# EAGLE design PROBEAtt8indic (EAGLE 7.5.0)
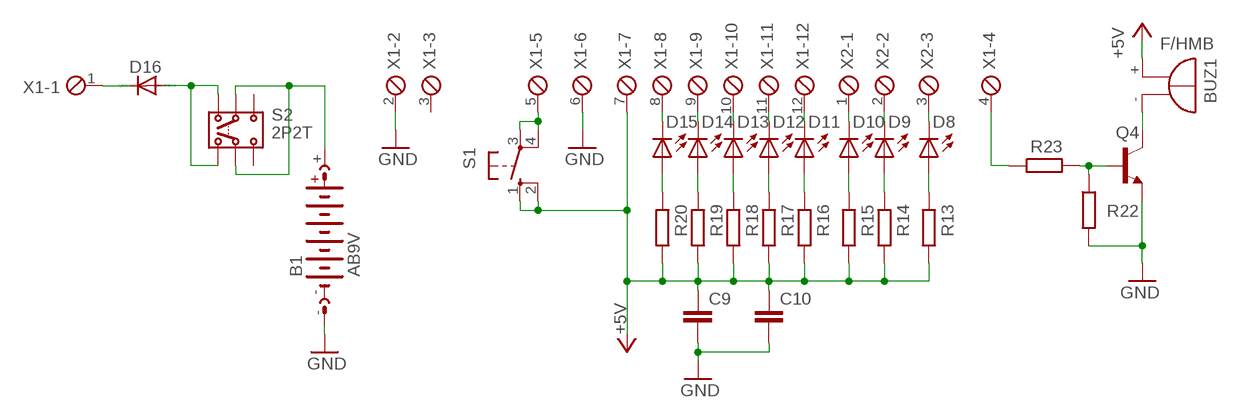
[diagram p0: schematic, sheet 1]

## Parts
B1  AB9V  [AB9V]
BUZ1  F/HMB  [F/HMB]
C9  C-EUC1206  [C1206]
C10  C-EUC1206  [C1206]
D8  LED5MM  [LED5MM]
D9  LED5MM  [LED5MM]
D10  LED5MM  [LED5MM]
D11  LED5MM  [LED5MM]
D12  LED5MM  [LED5MM]
D13  LED5MM  [LED5MM]
D14  LED5MM  [LED5MM]
D15  LED5MM  [LED5MM]
D16  1N4004  [DO41-10]
Q4  BC337  [TO92]
R13  R-EU_0204/7  [0204/7]
R14  R-EU_0204/7  [0204/7]
R15  R-EU_0204/7  [0204/7]
R16  R-EU_0204/7  [0204/7]
R17  R-EU_0204/7  [0204/7]
R18  R-EU_0204/7  [0204/7]
R19  R-EU_0204/7  [0204/7]
R20  R-EU_0204/7  [0204/7]
R22  R-EU_0204/7  [0204/7]
R23  R-EU_0204/7  [0204/7]
S1  10-XX  [B3F-10XX]
S2  2P2T  [2P2T]
X1  MPT12  [12POL254]
X2  MPT3  [3POL254]

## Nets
+5V: BUZ1.+ C9.1 C10.1 R13.1 R14.1 R15.1 R16.1 R17.1 R18.1 R19.1 R20.1 S1.1(S) S1.2(S1) X1.7
GND: B1.- C9.2 C10.2 Q4.1(E) R22.2 X1.2 X1.6
N$1: R23.1 X1.4
N$2: D8.K(C) X2.3
N$3: D9.K(C) X2.2
N$4: S1.3(P) S1.4(P1) X1.5
N$5: D10.K(C) X2.1
N$6: D16.C X1.1
N$7: D11.K(C) X1.12
N$8: D12.K(C) X1.11
N$9: Q4.2(B) R22.1 R23.2
N$10: D13.K(C) X1.10
N$11: D14.K(C) X1.9
N$12: D15.K(C) X1.8
N$13: D15.A R20.2
N$14: D14.A R19.2
N$15: D13.A R18.2
N$16: D12.A R17.2
N$17: D11.A R16.2
N$18: D10.A R15.2
N$19: D9.A R14.2
N$20: D16.A S2.1.1 S2.1.2
N$21: D8.A R13.2
N$22: B1.+ S2.2.1 S2.2.2
N$23: BUZ1.- Q4.3(C)
Unconnected: S2.3.1 S2.3.2 X1.3

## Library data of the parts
B1 = battery:AB9V: 9-V BATTERY CLIP
BUZ1 = buzzer:F/HMB: BUZZER; OC_FARNELL: unknown; OC_NEWARK: unknown
C9 C10 = rcl:C-EU: CAPACITOR, European symbol
D8-D15 = led:LED: LED
D16 = diode:1N4004: DIODE
Q4 = transistor:BC337: NPN TRANSISTOR
R13-R20 R22 R23 = rcl:R-EU_: RESISTOR, European symbol
S1 = switch-omron:10-XX: OMRON SWITCH; MPN: B3F-1000; OC_FARNELL: 176432; OC_NEWARK: 36M3542
S2 = switch:2P2T: SLIDE SWITCH 2P2T Part No. SS-22F05-G(A)4 Source: CANAL ELECTRONIC CO., LTD .. switsch.pdf
X1 = con-phoenix-254:MPT12: PHOENIX CONNECTOR; OC_FARNELL: unknown; OC_NEWARK: unknown
X2 = con-phoenix-254:MPT3: PHOENIX CONNECTOR; OC_FARNELL: unknown; OC_NEWARK: unknown

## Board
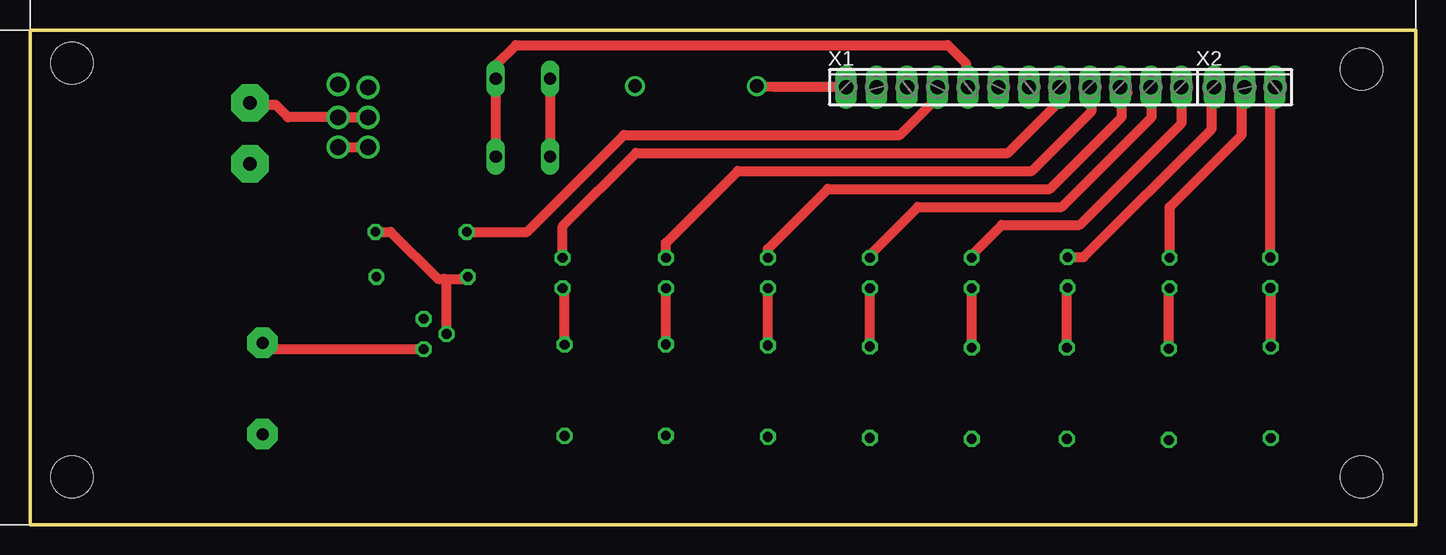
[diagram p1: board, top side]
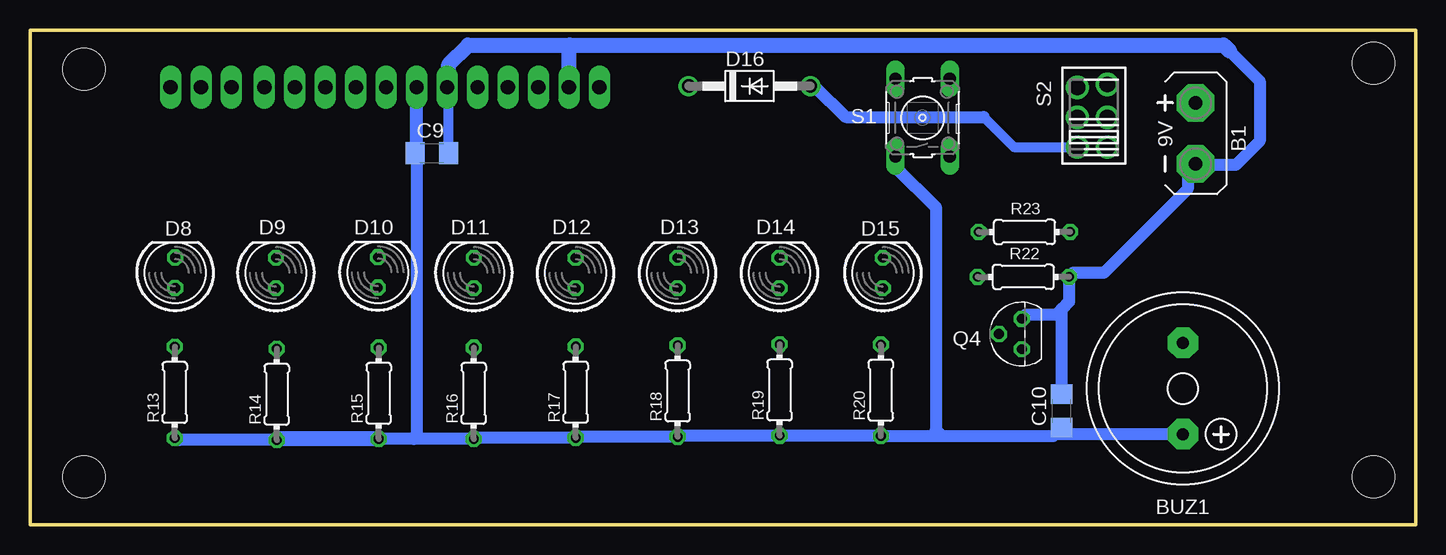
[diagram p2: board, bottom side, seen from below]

Size 115.5 x 41.25 mm. Coordinates in mm from the lower left corner, seen from the top.
Outline: 0,0 0,41.25 115.5,41.25 115.5,0 0,0
Copper layers (1*16): Top 0.035mm / dielectric 1.5mm / Bottom 0.035mm
Design rules "default": minimum track width 10mil, minimum drill 24mil, track to track 8mil, track to pad 8mil, pad to pad 8mil, via to via 8mil, smd to smd 8mil, copper to edge 40mil, drill to drill 8mil, minimum pad ring 10mil, minimum via ring 8mil, stop-mask expansion 4mil, vias tented up to drill 0mil, thermal gap 10mil
Holes 3.5 mm at 3.5,38.5 3.5,4 111,38 111,4

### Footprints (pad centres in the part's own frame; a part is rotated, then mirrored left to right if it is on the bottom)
AB9V = drill 1.118 pad 3.15 octagon: + 0,2.54; - 0,-2.54
F/HMB = drill 1.016 pad 2.54 octagon: + 3.81,0; - -3.81,0
C1206 = smd 1.6 x 1.8: 1 -1.4,0; 2 1.4,0
LED5MM = drill 0.813 octagon: A -1.27,0; K 1.27,0
DO41-10 = drill 1.118: A 5.08,0; C -5.08,0
TO92 = drill 0.813 octagon: 1 1.27,0; 2 0,1.905; 3 -1.27,0
0204/7 = drill 0.813 octagon: 1 -3.81,0; 2 3.81,0
B3F-10XX = drill 1.016 long: 1 -3.251,2.261; 2 3.251,2.261; 3 -3.251,-2.261; 4 3.251,-2.261
2P2T = drill 1.3 pad 1.93: 1.1 -2.492,1.38; 1.2 -2.492,-1.126; 2.1 0,1.38; 2.2 0,-1.126; 3.1 2.492,1.38; 3.2 2.746,-1.126
12POL254 = drill 1.2 long: 1 -13.97,0; 2 -11.43,0; 3 -8.89,0; 4 -6.35,0; 5 -3.81,0; 6 -1.27,0; 7 1.27,0; 8 3.81,0; 9 6.35,0; 10 8.89,0; 11 11.43,0; 12 13.97,0
3POL254 = drill 1.2 long: 1 -2.54,0; 2 0,0; 3 2.54,0

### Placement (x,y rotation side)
B1  18.33,32.65 0 bottom
BUZ1  19.39,11.36 270 bottom
C9  82,31 0 bottom
C10  29.5,9.5 90 bottom
D8  103.4,21.02 90 bottom
D9  95,21 90 bottom
D10  86.5,21.05 90 bottom
D11  78.5,21 90 bottom
D12  70.02,21 90 bottom
D13  61.52,21 90 bottom
D14  53.02,21 90 bottom
D15  44.4,21 90 bottom
D16  55.52,36.59 0 bottom
Q4  32.82,15.91 90 bottom
R13  103.43,11.04 90 bottom
R14  94.93,10.88 90 bottom
R15  86.43,10.97 90 bottom
R16  78.51,10.97 90 bottom
R17  70.01,11.06 90 bottom
R18  61.51,11.15 90 bottom
R19  53.01,11.24 90 bottom
R20  44.57,11.22 90 bottom
R22  32.69,20.68 0 bottom
R23  32.6,24.43 0 bottom
S1  41.09,33.95 90 bottom
S2  26.81,33.99 90 bottom
X1  82,36.5 0 top
X2  101.25,36.5 0 top

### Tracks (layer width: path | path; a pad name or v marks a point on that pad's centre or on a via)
+5V
  Top 0.813: S1.2 S1.1
  Bottom 0.813: C9.1 83.4,35.87 83.27,36
  Bottom 1.016: 39.5,7.41 R20.1 52.99,7.41 R19.1 61.42,7.43 R18.1 69.92,7.34 R17.1 78.42,7.25 R16.1 83.5,7.16 | 39.5,7.41 30.19,7.41 30.05,7.55 | 30.05,7.55 C10.1 | 83.5,7.16 R15.1 | 94.9,7.1 R14.1 103.09,7.07 R13.1 | S1.1 43.35,29.85 40,26.5 40,7.91 39.5,7.41 | X1.7 83.27,36 83.27,7.39 83.5,7.16 | BUZ1.+ 30.05,7.55
  Bottom 1.27: R15.1 94.84,7.16 R14.1
GND
  Bottom 0.813: C9.2 80.6,36.37 X1.6
  Bottom 1.016: 15.5,39.5 13,37 13,32 15,30 18.44,30 | 18.44,30 19,30 19,28 26,21 28.56,21 R22.2 28.88,18.62 29.5,18 | 18.44,30 B1.- | 29.5,18 30,17.5 32.5,17.5 Q4.1 | C10.2 29.5,18
  Bottom 1.27: 80.6,36.37 80.6,38.4 79,40 70.5,40 | 70.5,40 16,40 15.5,39.5 | X1.2 70.57,39.93 70.5,40
N$1
  Top 0.813: R23.1 41.43,24.43 49.5,32.5 72.5,32.5 76,36 76,36.15 X1.4
N$2
  Top 0.813: D8.K 103.4,36.11 X2.3
N$3
  Top 0.813: D9.K 95,26.5 101,32.5 101,36.25 X2.2
N$4
  Top 0.813: X1.5 78,36.69 78,38.5 76.5,40 40.5,40 38.83,38.33 S1.4 S1.3
N$5
  Top 0.813: D10.K 87.82,22.32 98.5,33 98.5,36.29 X2.1
N$6
  Top 0.813: X1.1 62.01,36.5 D16.C
N$7
  Top 0.813: D11.K 78.5,22.5 81,25 87.5,25 96,33.5 96,36.47 X1.12
N$8
  Top 0.813: D12.K 70.02,22.52 74,26.5 86,26.5 93.5,34 93.5,36.43 X1.11
N$9
  Top 0.813: R23.2 30.07,24.43 34,20.5 34.5,20.5 | 34.5,20.5 36.32,20.5 R22.1 | Q4.2 34.73,20.27 34.5,20.5
N$10
  Top 0.813: D13.K 61.52,23.02 66.5,28 85,28 91,34 91,35.5 91.5,36 91.39,36 X1.10
N$11
  Top 0.813: D14.K 53.02,23.52 59,29.5 83.5,29.5 88.5,34.5 88.5,36.35 X1.9
N$12
  Top 0.813: D15.K 44.4,24.9 50.5,31 81.5,31 85.5,35 85.5,36.19 X1.8
N$13
  Top 0.813: R20.2 44.57,19.56 D15.A
N$14
  Top 0.813: R19.2 D14.A
N$15
  Top 0.813: R18.2 D13.A
N$16
  Top 0.813: R17.2 D12.A
N$17
  Top 0.813: R16.2 D11.A
N$18
  Top 0.813: R15.2 86.43,19.71 D10.A
N$19
  Top 0.813: R14.2 94.93,19.66 D9.A
N$20
  Top 0.813: S2.1.2 S2.1.1
  Bottom 0.813: 36,34 33.5,31.5 S2.1.1
  Bottom 1.016: D16.A 50.09,36.59 47.5,34 36,34
N$21
  Top 0.813: R13.2 103.43,19.72 D8.A
N$22
  Top 0.813: S2.2.1 S2.2.2 21.51,33.99 20.5,35 18.52,35 B1.+
N$23
  Top 0.813: Q4.3 20.36,14.64 20,15 19.56,15 BUZ1.-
